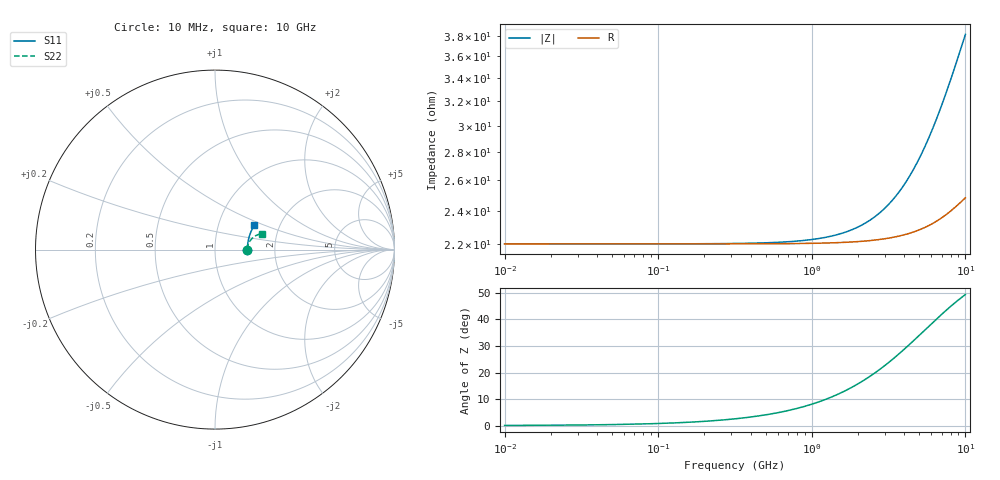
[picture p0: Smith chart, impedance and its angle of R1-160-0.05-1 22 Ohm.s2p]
!version-1
!date-03.2021
# MHz S RI R 50
!Freq ReS11 ImS11 ReS21 ImS21 ReS12 ImS12 ReS22 ImS22
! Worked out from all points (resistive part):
!   501 points, 10 MHz to 10 GHz, reference 50 ohm
!   read as one part in series: R = 22 ohm at 50 MHz
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10  0.1803 0.000164  0.8197 -0.000269  0.8197 -0.000269  0.1803 0.000133
50  0.1803 0.000819  0.8197 -0.00134  0.8197 -0.00134  0.1803 0.000663
410  0.1804 0.00672  0.8195 -0.011  0.8195 -0.011  0.1805 0.00543
830  0.1807 0.0136  0.8191 -0.0223  0.8191 -0.0223  0.181 0.011
1250  0.1811 0.0204  0.8183 -0.0335  0.8183 -0.0335  0.1819 0.0165
1690  0.1818 0.0276  0.8172 -0.0452  0.8172 -0.0452  0.1832 0.0222
2090  0.1826 0.034  0.816 -0.0558  0.816 -0.0558  0.1848 0.0273
2490  0.1835 0.0404  0.8144 -0.0663  0.8144 -0.0663  0.1866 0.0322
2910  0.1846 0.047  0.8126 -0.0772  0.8126 -0.0772  0.1889 0.0374
3350  0.186 0.0538  0.8103 -0.0886  0.8103 -0.0886  0.1916 0.0425
3710  0.1873 0.0593  0.8082 -0.0977  0.8082 -0.0977  0.194 0.0467
4110  0.1888 0.0654  0.8057 -0.1078  0.8057 -0.1078  0.197 0.0511
4530  0.1905 0.0716  0.8029 -0.1182  0.8029 -0.1182  0.2005 0.0555
5010  0.1926 0.0785  0.7993 -0.1299  0.7993 -0.1299  0.2047 0.0603
5850  0.1966 0.0902  0.7924 -0.1497  0.7924 -0.1497  0.2129 0.0679
6670  0.2009 0.101  0.785 -0.1683  0.785 -0.1683  0.2217 0.0743
7510  0.2056 0.1114  0.7769 -0.1865  0.7769 -0.1865  0.2313 0.0798
8350  0.2103 0.1211  0.7683 -0.2038  0.7683 -0.2038  0.2414 0.0841
8790  0.2128 0.1259  0.7637 -0.2125  0.7637 -0.2125  0.2469 0.0859
9230  0.2152 0.1305  0.759 -0.2209  0.759 -0.2209  0.2523 0.0874
9730  0.218 0.1354  0.7537 -0.2302  0.7537 -0.2302  0.2586 0.0887
10000  0.2194 0.138  0.7508 -0.2351  0.7508 -0.2351  0.2619 0.0892
